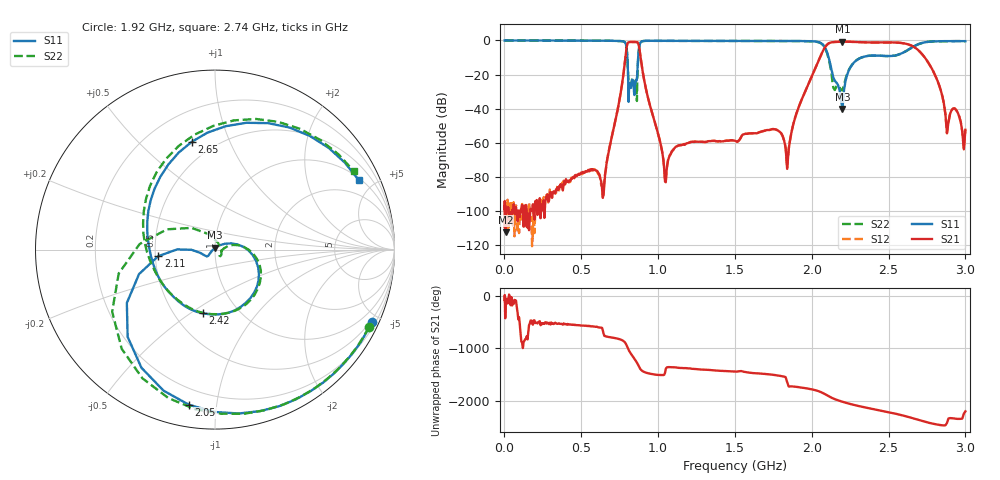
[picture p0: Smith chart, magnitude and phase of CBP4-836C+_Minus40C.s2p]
! Mini-Circuits
! S2P DATA File Format
! Type: BAND PASS FILTER
! Model: CBP4-836C+
! All S Parameters are in dB deg format
! TEST CONDITIONS: INPUT POWER = 0 dBm @ Temperature = -40deg C
! 636 Frequency points
# MHz S DB R 50
!FREQMAG(S11)PHS(S11)MAG(S21)PHS(S21)MAG(S12)PHS(S12)MAG(S22)PHS(S22)
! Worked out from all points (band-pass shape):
!   636 points, 1 MHz to 3 GHz, reference 50 ohm
!   highest |S21| = -0.72 dB at 2.2 GHz (marker M1); lowest = -112.4 dB at 8 MHz (marker M2)
!   |S21| within 3 dB of the highest: 795.8 MHz to 875.9 MHz (80.13 MHz wide, 9.59 % of centre); 2.088 GHz to 2.664 GHz (575.1 MHz wide, 24.2 % of centre)
!   lowest |S11| = -40.1 dB at 2.2 GHz (marker M3), VSWR 1.02, Z = 50.1 + j0.985 ohm
!   |S11| at or under -10 dB: 799.9 MHz to 870.1 MHz (70.28 MHz wide, 8.42 % of centre); 2.11 GHz to 2.324 GHz (213.5 MHz wide, 9.63 % of centre)
!   |S22| runs from -35.5 to 0.0 dB; largest |S21 - S12| = 0.017
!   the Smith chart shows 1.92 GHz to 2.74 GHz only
!   S11 on the Smith chart (normalised r, x): 1.92 GHz: 0.41, -4.51; 2.05 GHz: 0.11, -0.84; 2.11 GHz: 0.52, -0.04; 2.42 GHz: 0.69, -0.56; 2.65 GHz: 0.38, +0.73; 2.74 GHz: 1.10, +4.08
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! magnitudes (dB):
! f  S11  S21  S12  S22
! 1 MHz  0.0  -109.3  -95.5  0.0
! 8 MHz  0.0  -112.4  -99.5  0.0
! 505 MHz  -0.1  -77.9  -78.4  -0.1
! 650 MHz  -0.2  -84.5  -80.9  -0.2
! 787 MHz  -1.5  -10.1  -10.1  -1.5
! 807 MHz  -32.0  -1.1  -1.1  -24.3
! 861 MHz  -23.3  -1.0  -1.0  -33.2
! 872 MHz  -7.8  -2.2  -2.2  -8.2
! 1.005 GHz  -0.2  -56.3  -56.5  -0.2
! 1.05 GHz  -0.2  -83.1  -82.6  -0.2
! 1.505 GHz  -0.3  -58.9  -58.9  -0.3
! 1.84 GHz  -0.3  -75.2  -75.1  -0.3
! 1.92 GHz  -0.3  -37.9  -37.9  -0.3
! 2.01 GHz  -0.5  -19.1  -19.1  -0.6
! 2.05 GHz  -1.1  -10.7  -10.7  -1.2
! 2.11 GHz  -9.9  -1.7  -1.7  -10.7
! 2.2 GHz  -40.1  -0.7  -0.7  -29.2
! 2.42 GHz  -8.8  -1.2  -1.2  -8.9
! 2.51 GHz  -9.1  -1.1  -1.1  -9.1
! 2.65 GHz  -4.2  -3.1  -3.1  -4.3
! 2.74 GHz  -1.0  -10.5  -10.5  -1.0
! 3 GHz  -0.4  -52.3  -52.3  -0.4
